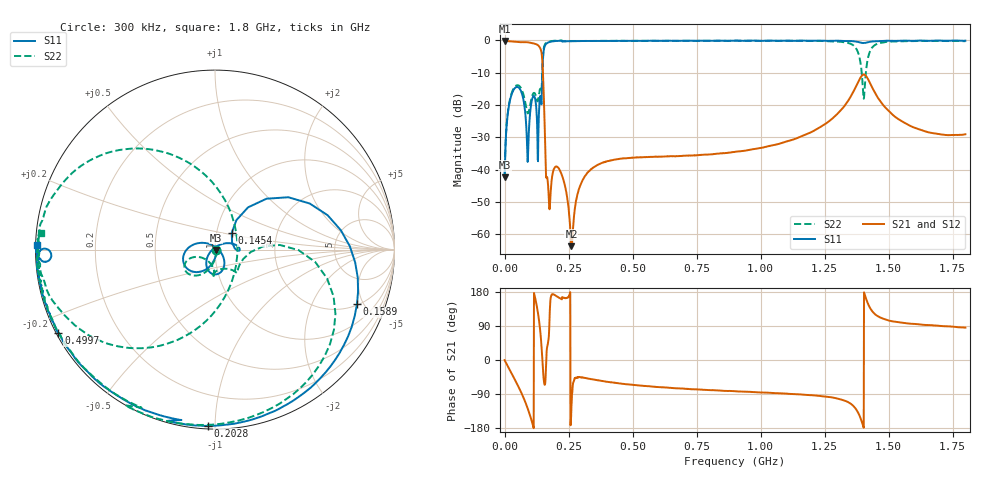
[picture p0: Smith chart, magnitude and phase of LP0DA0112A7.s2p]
!Agilent Technologies,E8358A,US41080443,A.07.50.56
!Agilent E8358A: A.07.50.56
!Date: Wednesday, February 06, 2019 13:32:06
!Correction: S11(Full 2 Port(1,2))
!S21(Full 2 Port(1,2))
!S12(Full 2 Port(1,2))
!S22(Full 2 Port(1,2))
!S2P File: Measurements: S11, S21, S12, S22:
# Hz S  dB  R 50
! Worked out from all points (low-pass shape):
!   1601 points, 300 kHz to 1.8 GHz, reference 50 ohm
!   highest |S21| = -0.13 dB at 300 kHz (marker M1); lowest = -63.7 dB at 261.3 MHz (marker M2)
!   |S21| within 3 dB of the highest: start of sweep to 142.8 MHz
!   lowest |S11| = -42.4 dB at 300 kHz (marker M3), VSWR 1.02, Z = 50.7 - j0.161 ohm
!   |S11| at or under -10 dB: start of sweep to 147.9 MHz
!   |S22| runs from -42.4 to 0.0 dB; largest |S21 - S12| = 0.0095
!   S11 on the Smith chart (normalised r, x): 300 kHz: 1.01, -0.00; 145.4 MHz: 1.18, +0.22; 158.9 MHz: 2.06, -4.46; 202.8 MHz: 0.02, -0.96; 499.7 MHz: 0.01, -0.25; 1.8 GHz: 0.00, +0.01
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300000  -42.37 -12.0  -0.13 -0.4  -0.07 -0.4  -42.40 -12.7
2.392106e7  -17.71 -117.4  -0.29 -30.7  -0.22 -30.8  -17.37 -112.8
6.553912e7  -15.92 -179.1  -0.51 -86.3  -0.44 -86.4  -14.95 -156.4
9.0285e7  -37.62 60.1  -0.56 -127.6  -0.49 -127.6  -22.51 -131.5
1.094068e8  -17.76 -75.3  -0.83 -168.5  -0.76 -168.5  -16.86 -92.3
1.319031e8  -30.12 50.5  -1.56 118.1  -1.49 118.0  -18.22 -60.3
1.454008e8  -17.62 44.9  -4.27 26.3  -4.20 26.3  -13.99 -3.8
1.588986e8  -1.44 -21.1  -33.14 -61.3  -33.05 -61.1  -1.07 -52.1
1.712715e8  -0.58 -55.1  -46.31 50.7  -46.21 50.3  -0.39 -79.1
2.027662e8  -0.15 -92.3  -39.06 168.4  -38.96 168.6  -0.05 -109.1
2.612565e8  -0.20 -116.0  -63.74 -124.6  -64.28 -130.3  -0.18 -127.3
3.006249e8  -0.17 -126.6  -44.06 -45.9  -43.96 -45.7  -0.17 -136.2
4.997168e8  -0.10 -151.9  -36.37 -65.7  -36.28 -65.4  -0.09 -158.1
6.009499e8  -0.11 -158.4  -36.03 -71.4  -35.92 -71.5  -0.09 -164.0
9.0015e8  -0.05 -169.1  -34.53 -82.6  -34.47 -82.5  -0.07 -174.7
1.200475e9  -0.10 -175.5  -28.30 -92.9  -28.26 -92.9  -0.16 174.4
1.343326e9  -0.18 -178.7  -18.53 -111.6  -18.47 -111.7  -0.79 153.6
1.38157e9  -0.47 179.7  -12.79 -139.7  -12.78 -139.6  -3.90 120.3
1.402941e9  -0.80 -177.9  -10.56 -178.9  -10.51 -179.0  -18.04 2.0
1.427687e9  -0.39 -176.0  -13.22 137.2  -13.21 137.2  -3.31 -126.5
1.5008e9  -0.07 -178.2  -21.89 104.2  -21.85 104.3  -0.35 -165.2
1.8e9  -0.05 178.5  -29.06 85.4  -29.03 85.4  -0.23 174.4
